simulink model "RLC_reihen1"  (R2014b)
settings: Solver=ode45  StartTime=0.0  StopTime=10.0  RelTol=1e-3
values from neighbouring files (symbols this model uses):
  ampl_ug = 2    [RLC_reihen_1.m]    (also in RLC_reihen_3.m; RLC_reihen_4.m)
  C = [0 1 0 0;0 0 0 1]    [impuls_antw_zustand_1.m]    (also in impuls_antwort_1.m = 1e-07; impuls_antwort_2.m = 1e-07; impuls_antwort_3.m = 1e-07; impuls_antwort_4.m = 1e-07)
  f_ug = 1000    [RLC_reihen_1.m]    (also in RLC_reihen_3.m; RLC_reihen_4.m)
  i0 = 0    [RLC_reihen_1.m]    (also in RLC_reihen_3.m; RLC_reihen_4.m)
  L = 0.01    [impuls_antwort_1.m]    (also in impuls_antwort_2.m; impuls_antwort_3.m; impuls_antwort_4.m; RLC_reihen_1.m)
  phi_ug = pi/3    (= 1.0471975512)    [RLC_reihen_1.m]    (also in RLC_reihen_3.m; RLC_reihen_4.m)
  R = 50    [impuls_antwort_1.m]    (also in impuls_antwort_2.m; impuls_antwort_3.m; impuls_antwort_4.m; RLC_reihen_1.m)
  uc0 = -2    [RLC_reihen_1.m]    (also in RLC_reihen_3.m; RLC_reihen_4.m)

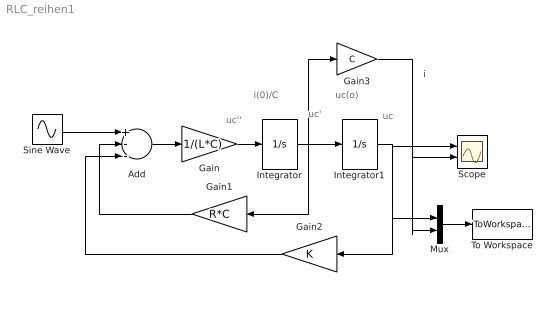
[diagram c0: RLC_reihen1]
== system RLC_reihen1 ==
  note: i
  note: uc(o)
  note: i(0)/C
  note: uc''
  note: uc
  note: uc'
  Add : Sum  Inputs=+--
  Gain : Gain  Gain=1/(L*C)
  Gain1 : Gain  Gain=R*C
  Gain2 : Gain
  Gain3 : Gain  Gain=C
  Integrator : Integrator  InitialCondition=i0/C
  Integrator1 : Integrator  InitialCondition=uc0
  Mux : Mux  Inputs=2
  Scope : Scope  NumInputPorts=2
  Sine Wave : Sin  Amplitude=ampl_ug  Frequency=2*pi*f_ug  Phase=phi_ug  SampleTime=0
  To Workspace : ToWorkspace  VariableName=simout  SaveFormat=Timeseries  SampleTime=-1
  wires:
  Sine Wave/1 -> Add/1
  Add/1 -> Gain/1
  Gain/1 -> Integrator/1
  Integrator/1 -> Gain1/1, Integrator1/1, Gain3/1
  Gain1/1 -> Add/2
  Gain2/1 -> Add/3
  Integrator1/1 -> Scope/1, Mux/1, Gain2/1
  Gain3/1 -> Scope/2, Mux/2
  Mux/1 -> To Workspace/1
